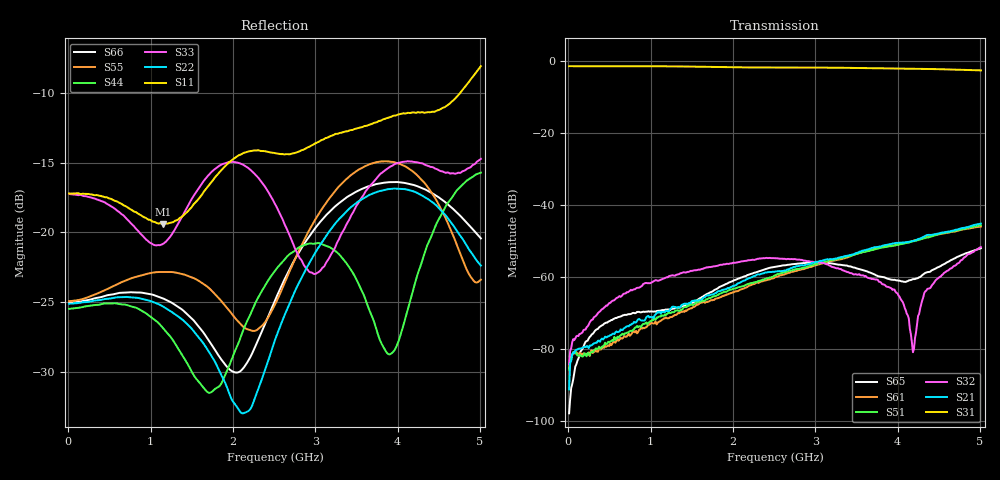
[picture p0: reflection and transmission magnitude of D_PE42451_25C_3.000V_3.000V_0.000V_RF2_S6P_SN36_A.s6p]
! Device ID: PE42451
! Serial: 36
! Insertion: A
! Temp: 25C
! VDD: 3.000
! Control_Hi: 100.000
! Control_Lo: 0.000
! Logic State: RF2
! Port 1: RFC
! Port 2: RF1
! Port 3: RF2
! Port 4: RF3
! Port 5: RF4
! Port 6: RF5
! V1 = 0.00
! V2 = 3.00
! V3 = 0.00
! V4 = 0.00
! IDD: 1.331820e-05
#  Hz  S  RI  R  50
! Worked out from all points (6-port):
!   401 points, 10 MHz to 5.01 GHz, reference 50 ohm
!   strongest paths, dB at 10 MHz, 1.26 GHz, 2.51 GHz, 3.76 GHz, 5.01 GHz:
!     S31: -1.4, -1.5, -1.8, -2.0, -2.6
!     S21: -91.1, -68.2, -58.4, -51.6, -45.1
!     S32: -84.1, -59.5, -54.7, -60.8, -51.6
!     S51: -85.7, -69.7, -59.5, -52.0, -45.5
!     S61: -85.2, -71.0, -60.0, -51.8, -45.9
!     S65: -97.8, -68.8, -57.1, -59.7, -51.9
!   lowest |S11| = -19.4 dB at 1.147 GHz (marker M1), VSWR 1.24, Z = 57.5 - j8.74 ohm
!   |S11| at or under -10 dB: start of sweep to 4.759 GHz
